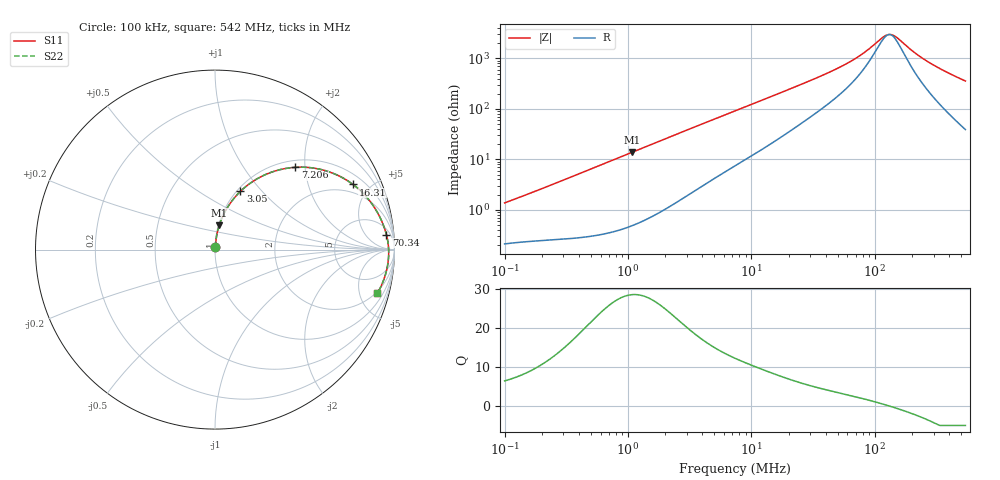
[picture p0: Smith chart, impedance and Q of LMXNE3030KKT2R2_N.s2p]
! LMXNE3030KKT2R2_N  S-PARAMETER MODEL  ( General Type )
! Model Generated by TAIYO YUDEN Corporation (http://www.ty-top.com)
! Version 1.0
! TAIYO YUDEN Control No. 191023NI43SB-FBB
! Copyright(c) 2019 TAIYO YUDEN CO.,LTD. All Rights Reserved.
! Product Description (link to TY-COMPAS)
! https://ds.yuden.co.jp/TYCOMPAS/or/detail?pn=LMXNE3030KKT2R2MN&u=M
! Products Name : Inductors
! Characteristics :
!  Inductance : 2.2 uH , SRF(min) : 86 MHz , DC Resistance(max) : 0.0996 Ohm
!  Rated Current : Saturation :1300 mA , Temp Rise : 1300 mA
!  Case Size : 3.0 x 3.0 / 0.118 x 0.118 [mm/inch] , Thickness : 1 / 0.039 [mm/inch]
!  (Conditions: Temperature = 25 degC , DC Bias Current/Voltage = 0A / 0V)
! External Node Assignments :
!  1  o---GGG---o  2
! GND o---------o GND
! Frequency Range : 0.1MHz  -  542.002916MHz  [ 402 STEP ]
# MHz S RI R 50
! Freq[MHz].  S11 Real  S11 Imag  S21 Real  S21 Imag  S12 Real  S12 Imag  S22 Real  S22 Imag
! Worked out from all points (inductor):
!   401 points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, 100 kHz to 542 MHz, reference 50 ohm
!   read as one part in series: L = 2.11 uH near 104.4 kHz
!   highest Q = 28.6 at 1.087 MHz (marker M1), where L = 2.04 uH
!   self-resonance near 130.7 MHz
!   S11 on the Smith chart (normalised r, x): 100 kHz: 1.00, +0.03; 3.05 MHz: 1.04, +0.77; 7.206 MHz: 1.14, +1.78; 16.31 MHz: 1.50, +3.92; 70.34 MHz: 9, +19; 542 MHz: 1.78, -7.09
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0.1  0.00228 0.0135  0.9977 -0.0135  0.9977 -0.0135  0.00228 0.0135
0.422129  0.00573 0.0538  0.9943 -0.0538  0.9943 -0.0538  0.00573 0.0538
1.08689  0.0235 0.1351  0.9765 -0.1351  0.9765 -0.1351  0.0235 0.1351
1.78193  0.0565 0.2125  0.9435 -0.2125  0.9435 -0.2125  0.0565 0.2125
3.04976  0.1419 0.3248  0.8581 -0.3248  0.8581 -0.3248  0.1419 0.3248
4.588077  0.2619 0.4091  0.7381 -0.4091  0.7381 -0.4091  0.2619 0.4091
7.205528  0.4471 0.4584  0.5529 -0.4584  0.5529 -0.4584  0.4471 0.4584
7.362085  0.4567 0.4589  0.5433 -0.4589  0.5433 -0.4589  0.4567 0.4589
10.60952  0.6164 0.4394  0.3836 -0.4394  0.3836 -0.4394  0.6164 0.4394
16.30782  0.7689 0.363  0.2311 -0.363  0.2311 -0.363  0.7689 0.363
22.03363  0.842 0.2956  0.158 -0.2956  0.158 -0.2956  0.842 0.2956
31.0775  0.8963 0.2217  0.1037 -0.2217  0.1037 -0.2217  0.8963 0.2217
49.86734  0.9384 0.1358  0.0616 -0.1358  0.0616 -0.1358  0.9384 0.1358
70.33577  0.9551 0.0835  0.0449 -0.0835  0.0449 -0.0835  0.9551 0.0835
87.20197  0.9616 0.0537  0.0384 -0.0537  0.0384 -0.0537  0.9616 0.0537
115.3138  0.9665 0.0165  0.0335 -0.0165  0.0335 -0.0165  0.9665 0.0165
131.1872  0.9676 -0.000446  0.0324 0.000446  0.0324 0.000446  0.9676 -0.000446
149.2455  0.9679 -0.0176  0.0321 0.0176  0.0321 0.0176  0.9679 -0.0176
210.5045  0.9648 -0.0657  0.0352 0.0657  0.0352 0.0657  0.9648 -0.0657
278.3662  0.9573 -0.1097  0.0427 0.1097  0.0427 0.1097  0.9573 -0.1097
392.6237  0.9381 -0.1734  0.0619 0.1734  0.0619 0.1734  0.9381 -0.1734
542.0029  0.9042 -0.2446  0.0958 0.2446  0.0958 0.2446  0.9042 -0.2446
